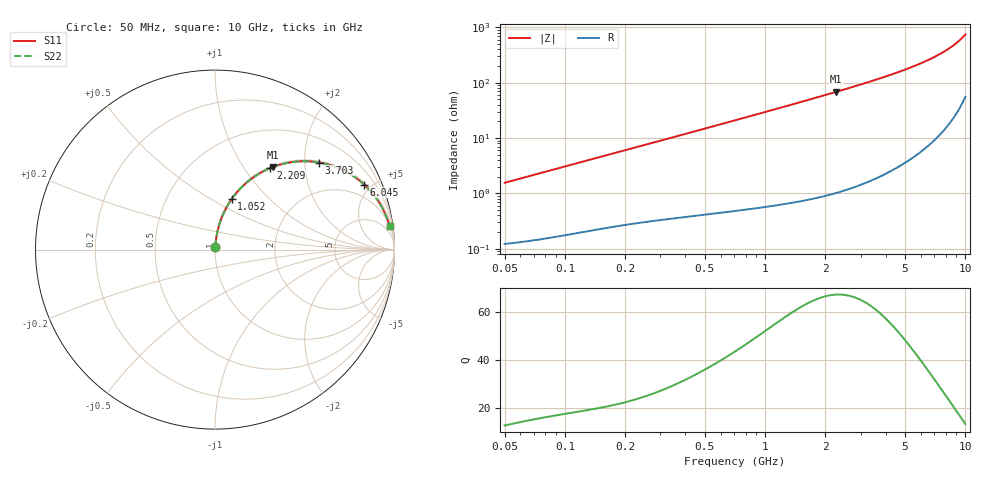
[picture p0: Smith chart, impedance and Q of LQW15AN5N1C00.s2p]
!Murata Part Number: LQW15AN5N1C00
!These Parameters are Measured in Series Mode Connection
!  o--[Z]--o
!Port1  Port2
!  o-------o
!Freq. Start=50[MHz] Stop=10[GHz], 401[Steps]
# Hz S RI R 50
!Freq.(Hz)	S 11(Real)	S 11(Imag)	S 21(Real)	S 21(Imag)	S 12(Real)	S 12(Imag)	S 22(Real)	S 22(Imag)
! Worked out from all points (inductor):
!   401 points, 50 MHz to 10 GHz, reference 50 ohm
!   read as one part in series: L = 4.91 nH near 51.34 MHz
!   highest Q = 67.2 at 2.268 GHz (marker M1), where L = 4.8 nH
!   S11 on the Smith chart (normalised r, x): 50 MHz: 1.00, +0.03; 1.052 GHz: 1.01, +0.62; 2.209 GHz: 1.02, +1.33; 3.703 GHz: 1.04, +2.36; 6.045 GHz: 1.12, +4.53; 10 GHz: 2, +15
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5e7  0.00146 0.0154  0.9985 -0.0154  0.9985 -0.0154  0.00146 0.0154
1.214486e8  0.00333 0.0368  0.9967 -0.0368  0.9967 -0.0368  0.00333 0.0368
1.956524e8  0.00607 0.0583  0.9939 -0.0583  0.9939 -0.0583  0.00607 0.0583
2.949953e8  0.0108 0.0866  0.9892 -0.0866  0.9892 -0.0866  0.0108 0.0866
4.689809e8  0.0226 0.135  0.9774 -0.135  0.9774 -0.135  0.0226 0.135
7.071068e8  0.0458 0.1979  0.9542 -0.1979  0.9542 -0.1979  0.0458 0.1979
1.052113e9  0.0921 0.28  0.9079 -0.28  0.9079 -0.28  0.0921 0.28
1.353197e9  0.1422 0.341  0.8578 -0.341  0.8578 -0.341  0.1422 0.341
1.717543e9  0.2107 0.4001  0.7893 -0.4001  0.7893 -0.4001  0.2107 0.4001
2.209055e9  0.309 0.4547  0.691 -0.4547  0.691 -0.4547  0.309 0.4547
2.268358e9  0.3209 0.4595  0.6791 -0.4595  0.6791 -0.4595  0.3209 0.4595
2.917498e9  0.447 0.4896  0.553 -0.4896  0.553 -0.4896  0.447 0.4896
3.286879e9  0.5128 0.492  0.4872 -0.492  0.4872 -0.492  0.5128 0.492
3.703027e9  0.58 0.4853  0.42 -0.4853  0.42 -0.4853  0.58 0.4853
4.171863e9  0.6468 0.4691  0.3532 -0.4691  0.3532 -0.4691  0.6468 0.4691
5.088839e9  0.7516 0.4216  0.2484 -0.4216  0.2484 -0.4216  0.7516 0.4216
6.045081e9  0.8308 0.3624  0.1692 -0.3624  0.1692 -0.3624  0.8308 0.3624
6.993273e9  0.8864 0.3021  0.1136 -0.3021  0.1136 -0.3021  0.8864 0.3021
7.983737e9  0.9268 0.2413  0.0732 -0.2413  0.0732 -0.2413  0.9268 0.2413
8.876195e9  0.9521 0.1896  0.0479 -0.1896  0.0479 -0.1896  0.9521 0.1896
9.738562e9  0.9689 0.1429  0.0311 -0.1429  0.0311 -0.1429  0.9689 0.1429
1e10  0.9728 0.1294  0.0272 -0.1294  0.0272 -0.1294  0.9728 0.1294
